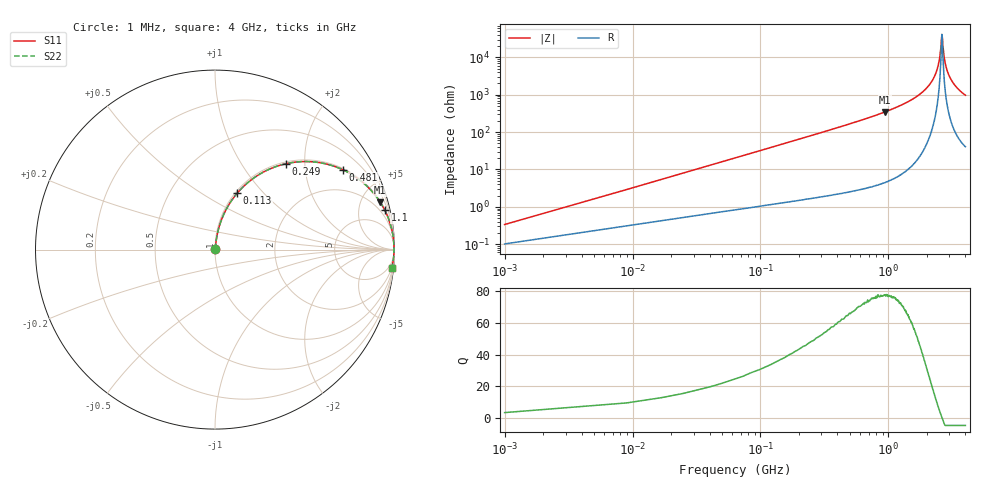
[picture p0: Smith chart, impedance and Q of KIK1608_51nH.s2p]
!version-2
!date-01.2022
!Series
# MHz S RI R 50
!Freq ReS11 ImS11 ReS21 ImS21 ReS12 ImS12 ReS22 ImS22
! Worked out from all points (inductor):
!   501 points, 1 MHz to 4 GHz, reference 50 ohm
!   read as one part in series: L = 51 nH near 17 MHz
!   highest Q = 77.6 at 945 MHz (marker M1), where L = 58.6 nH
!   self-resonance near 2.62 GHz
!   S11 on the Smith chart (normalised r, x): 1 MHz: 1.00, +0.01; 113 MHz: 1.02, +0.73; 249 MHz: 1.03, +1.61; 481 MHz: 1.05, +3.19; 1.1 GHz: 1.11, +8.61; 4 GHz: 2, -19
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1  0.00105 0.0032  0.999 -0.0032  0.999 -0.0032  0.00105 0.0032
25  0.0115 0.0788  0.9885 -0.0788  0.9885 -0.0788  0.0115 0.0788
33  0.0168 0.1034  0.9832 -0.1034  0.9832 -0.1034  0.0168 0.1034
65  0.049 0.1966  0.951 -0.1966  0.951 -0.1966  0.049 0.1966
113  0.1238 0.3144  0.8762 -0.3144  0.8762 -0.3144  0.1238 0.3144
249  0.3955 0.4787  0.6045 -0.4787  0.6045 -0.4787  0.3955 0.4787
481  0.7149 0.4438  0.2851 -0.4438  0.2851 -0.4438  0.7149 0.4438
673  0.8386 0.3611  0.1614 -0.3611  0.1614 -0.3611  0.8386 0.3611
945  0.9208 0.2637  0.0792 -0.2637  0.0792 -0.2637  0.9208 0.2637
1100  0.9462 0.2192  0.0538 -0.2192  0.0538 -0.2192  0.9462 0.2192
1335  0.9687 0.167  0.0313 -0.167  0.0313 -0.167  0.9687 0.167
2010  0.9938 0.0638  0.00621 -0.0638  0.00621 -0.0638  0.9938 0.0638
2410  0.9973 0.0204  0.00269 -0.0204  0.00269 -0.0204  0.9973 0.0204
2530  0.9976 0.00884  0.00244 -0.00884  0.00244 -0.00884  0.9976 0.00884
2620  0.9976 2.73e-05  0.00244 -2.73e-05  0.00244 -2.73e-05  0.9976 2.73e-05
2650  0.9975 -0.00213  0.00246 0.00213  0.00246 0.00213  0.9975 -0.00213
2670  0.9975 -0.00426  0.00249 0.00426  0.00249 0.00426  0.9975 -0.00426
2740  0.9973 -0.0106  0.00265 0.0106  0.00265 0.0106  0.9973 -0.0106
2860  0.9969 -0.0207  0.00309 0.0207  0.00309 0.0207  0.9969 -0.0207
3060  0.9958 -0.0367  0.00424 0.0367  0.00424 0.0367  0.9958 -0.0367
3335  0.9935 -0.057  0.00651 0.057  0.00651 0.057  0.9935 -0.057
4000  0.9853 -0.1011  0.0147 0.1011  0.0147 0.1011  0.9853 -0.1011
